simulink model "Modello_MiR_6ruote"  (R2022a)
settings: Solver=VariableStepAuto  StartTime=0.0  StopTime=time_v(end,1)  RelTol=1e-3
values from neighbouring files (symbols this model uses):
  a = 0.250    (= 0.25)    [Modello_MiR_6ruote_script.m]    (also in Modello_MiR_2ruote_script.m; Modello_MiR_6ruote_validato_script.m; Modello_MiR_UR_script.m)
  Att_C = 0.005    [Modello_MiR_6ruote_script.m]
  b = 0.1875    [Modello_MiR_6ruote_script.m]    (also in Modello_MiR_2ruote_script.m; Modello_MiR_6ruote_validato_script.m; Modello_MiR_UR_script.m)
  b_caster = 0.07    [Modello_MiR_6ruote_script.m]    (also in Modello_MiR_2ruote_script.m; Modello_MiR_6ruote_validato_script.m; Modello_MiR_UR_script.m)
  bd = 0.205    [Modello_MiR_6ruote_script.m]    (also in Modello_MiR_2ruote_script.m; Modello_MiR_6ruote_validato_script.m; Modello_MiR_UR_script.m)
  F23fun = @(u) (mv*9.801/4)-u(7)    [Modello_MiR_6ruote_script.m]    (also in Modello_MiR_6ruote_validato_script.m = @(u) (mv*9.801/4)-(mv*h*u(5)+(mv*9.801/4)*(2*a-b_caster*(cos)
  F43fun = @(u) (1/(2*bd))*(mv*u(6)*h+u(7)*(2*bd-b_caster*(sin(u(3))+sin(u(4))))+u(8)*(2*bd-b_caster*(sin(u(1))+sin(u(2)))))    [Modello_MiR_6ruote_script.m]    (also in Modello_MiR_6ruote_validato_script.m = @(u) (1/(2*bd))*(mv*u(6)*h+((mv*h*u(5)+(mv*9.801/4)*(2*a-b_c)
  F63fun = @(u) (mv*h*u(5)+(mv*9.801/4)*(2*a-b_caster*(cos(u(1))+cos(u(2)))))/(4*a-b_caster*(cos(u(1))+cos(u(2)))+b_caster*(cos(u(3))+cos(u(4))))    [Modello_MiR_6ruote_script.m]    (also in Modello_MiR_6ruote_validato_script.m)
  fm_fun = @(u) (u <= -am2 | u >= am2)*0 + (u > -am2 && u <= -am1)*(- u * Mza/(am2 -am1) - Mza * am2/(am2 -am1)) +           + (u > -am1 && u <= am1)*(Mza*u/ am1) + (u > am1 && u < am2)*(Mza * u/(am1 -am2) - Mza * am2/(am1 - am2))    [Modello_MiR_6ruote_script.m]    (also in Modello_MiR_6ruote_validato_script.m = @(u) (u <= -am2 || u >= am2) * 0 + (u > -am2 && u <= -am1) *; Modello_MiR_UR_script.m = @(u) (u <= -am2 || u >= am2) * 0 + (u > -am2 && u <= -am1) *)
  Icw_1 = 1/2 * mcw * rc^2    (= 0.002004225735)    [Modello_MiR_6ruote_script.m]    (also in Modello_MiR_2ruote_script.m; Modello_MiR_6ruote_validato_script.m; Modello_MiR_UR_script.m)
  Icw_2 = 1/12 * mcw * ec^2 + 1/4 * mcw * rc^2    (= 0.00104098243873)    [Modello_MiR_6ruote_script.m]    (also in Modello_MiR_2ruote_script.m; Modello_MiR_6ruote_validato_script.m; Modello_MiR_UR_script.m)
  Idw_1 = 1/2 * mdw * rd^2    (= 0.00551836278784)    [Modello_MiR_6ruote_script.m]    (also in Modello_MiR_2ruote_script.m; Transfer_Function_Gol_Gcl.m = Inertia_vect(jj,1); Modello_MiR_6ruote_validato_script.m; Modello_MiR_UR_script.m)
  iMax = 20.7*1.1    (= 22.77)    [Modello_MiR_6ruote_script.m]    (also in Modello_MiR_2ruote_script.m; Modello_MiR_6ruote_validato_script.m; Modello_MiR_UR_script.m)
  Iv = mv * (l^2 + w^2)  / 12    (= 6.75343333333)    [Modello_MiR_6ruote_script.m]    (also in Modello_MiR_2ruote_script.m; Modello_MiR_6ruote_validato_script.m = 8.95033333333; Modello_MiR_UR_script.m)
  Kc = 0.15    [Modello_MiR_6ruote_script.m]    (also in Modello_MiR_2ruote_script.m; Modello_MiR_6ruote_validato_script.m; Modello_MiR_UR_script.m)
  Ki_i = 1    [Modello_MiR_6ruote_script.m]    (also in Modello_MiR_2ruote_script.m; Modello_MiR_6ruote_validato_script.m; Modello_MiR_UR_script.m)
  Ki_v = 1    [Modello_MiR_6ruote_script.m]    (also in Modello_MiR_2ruote_script.m; Modello_MiR_6ruote_validato_script.m; Modello_MiR_UR_script.m)
  kk = 0.00005    (= 5e-05)    [Modello_MiR_6ruote_script.m]    (also in Modello_MiR_2ruote_script.m; Modello_MiR_6ruote_validato_script.m; Modello_MiR_UR_script.m)
  Kp_i = 5    [Modello_MiR_6ruote_script.m]    (also in Modello_MiR_2ruote_script.m; Modello_MiR_6ruote_validato_script.m; Modello_MiR_UR_script.m)
  Kp_v = 5    [Modello_MiR_6ruote_script.m]    (also in Modello_MiR_2ruote_script.m; Modello_MiR_6ruote_validato_script.m; Modello_MiR_UR_script.m)
  kv = 1.5e-6    (= 1.5e-06)    [Modello_MiR_6ruote_script.m]    (also in Modello_MiR_2ruote_script.m; Modello_MiR_6ruote_validato_script.m; Modello_MiR_UR_script.m)
  L = R * tauE    (= 0.00181134822805)    [Modello_MiR_6ruote_script.m]    (also in Modello_MiR_2ruote_script.m; Modello_MiR_6ruote_validato_script.m; Modello_MiR_UR_script.m)
  mcw = rc^2 * pi * ec * rhopoliu + 1    (= 1.02616357632)    [Modello_MiR_6ruote_script.m]    (also in Modello_MiR_2ruote_script.m; Modello_MiR_6ruote_validato_script.m; Modello_MiR_UR_script.m)
  mv = 83    [Modello_MiR_6ruote_script.m]    (also in Modello_MiR_2ruote_script.m; Modello_MiR_6ruote_validato_script.m = 110; Modello_MiR_UR_script.m)
  Psi_start = pi/2    (= 1.57079632679)    [Modello_MiR_6ruote_script.m]    (also in Modello_MiR_6ruote_validato_script.m = psi_mir(1,1); Modello_MiR_UR_script.m = psi_mir(1,1))
  R = velMax * TorqueMax / (iMax)^2    (= 1.81134822805)    [Modello_MiR_6ruote_script.m]    (also in Modello_MiR_2ruote_script.m; Modello_MiR_6ruote_validato_script.m; Modello_MiR_UR_script.m)
  rap_rid = 10.167    [Modello_MiR_6ruote_script.m]    (also in Modello_MiR_2ruote_script.m; Modello_MiR_6ruote_validato_script.m; Modello_MiR_UR_script.m)
  rc = 0.125/2    (= 0.0625)    [Modello_MiR_6ruote_script.m]    (also in Modello_MiR_2ruote_script.m; Modello_MiR_6ruote_validato_script.m; Modello_MiR_UR_script.m)
  rd = 0.1    [Modello_MiR_6ruote_script.m]    (also in Modello_MiR_2ruote_script.m; Modello_MiR_6ruote_validato_script.m; Modello_MiR_UR_script.m)
  Sx = spline(x ,fl_fun(x),zx)    [Modello_MiR_6ruote_script.m]
  Sy = spline(x ,ft_fun(x),zy)    [Modello_MiR_6ruote_script.m]
  VaMax = Kc * velMax    (= 41.2443991527)    [Modello_MiR_6ruote_script.m]    (also in Modello_MiR_2ruote_script.m; Modello_MiR_6ruote_validato_script.m; Modello_MiR_UR_script.m)
  X_start = input('Inserire coordinata x iniziale')    [Modello_MiR_6ruote_script.m]    (also in Modello_MiR_2ruote_script.m; Modello_MiR_6ruote_validato_script.m = traj(1,1); Modello_MiR_UR_script.m = traj(1,1))
  Y_start = input('Inserire coordinata y iniziale')    [Modello_MiR_6ruote_script.m]    (also in Modello_MiR_2ruote_script.m; Modello_MiR_6ruote_validato_script.m = traj(1,2); Modello_MiR_UR_script.m = traj(1,2))
  zx = linspace(inferior,superi,10001)    [Modello_MiR_6ruote_script.m]
  zy = linspace(inferior,superi,10001)    [Modello_MiR_6ruote_script.m]
libraries: slpidlib x4
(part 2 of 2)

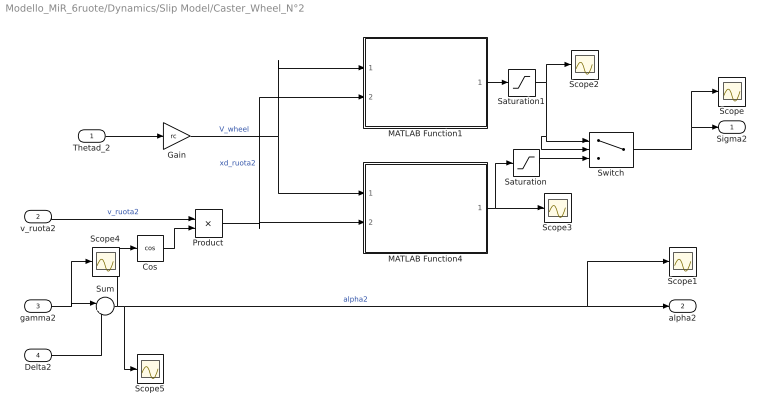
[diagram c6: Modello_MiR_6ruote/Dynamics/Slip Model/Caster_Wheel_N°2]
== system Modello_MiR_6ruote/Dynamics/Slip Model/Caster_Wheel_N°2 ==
  Thetad_2 : Inport
  v_ruota2 : Inport  Port=2
  gamma2 : Inport  Port=3
  Delta2 : Inport  Port=4
  Cos : Trigonometry  Operator=cos
  Gain : Gain  Gain=rc
  MATLAB Function1 : MATLAB Function  TreatAsAtomicUnit=on
  MATLAB Function4 : MATLAB Function  TreatAsAtomicUnit=on
  Product : Product
  Saturation : Saturate  UpperLimit=1  LowerLimit=-1
  Saturation1 : Saturate  UpperLimit=1  LowerLimit=-1
  Scope{,1..5} (6 alike) : Scope
  Sum : Sum  Inputs=|+-
  Switch : Switch
  Sigma2 : Outport
  alpha2 : Outport  Port=2
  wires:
  Thetad_2/1 -> Gain/1
  gamma2/1 -> Scope4/1, Sum/1
  Gain/1 -> MATLAB Function4/1(v_wheel), MATLAB Function1/1(v_wheel)  "V_wheel"
  Switch/1 -> Scope/1, Sigma2/1
  MATLAB Function1/1(Fc_pos_out) -> Saturation1/1
  MATLAB Function4/1(Fc_neg_out) -> Saturation/1, Scope3/1
  Product/1 -> MATLAB Function1/2(xd_ruota2), MATLAB Function4/2(xd_ruota2)  "xd_ruota2"
  v_ruota2/1 -> Product/1  "v_ruota2"
  Cos/1 -> Product/2
  Delta2/1 -> Sum/2
  Sum/1 -> Cos/1, Scope1/1, alpha2/1, Scope5/1  "alpha2"
  Saturation1/1 -> Scope2/1, Switch/2, Switch/1
  Saturation/1 -> Switch/3

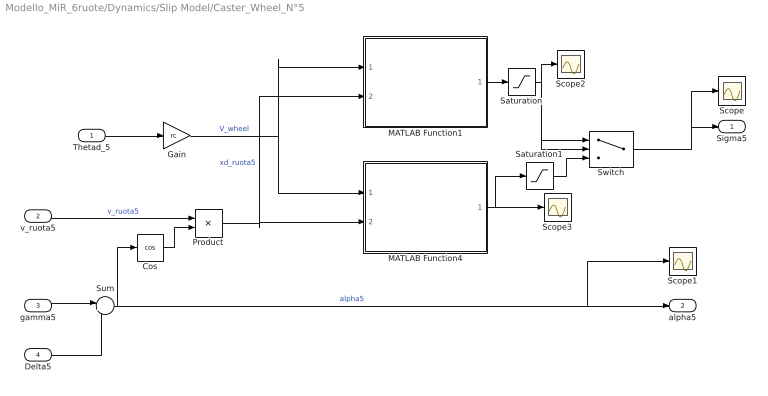
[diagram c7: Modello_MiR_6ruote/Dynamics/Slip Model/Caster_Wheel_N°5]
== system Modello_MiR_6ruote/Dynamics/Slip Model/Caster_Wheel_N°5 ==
  Thetad_5 : Inport
  v_ruota5 : Inport  Port=2
  gamma5 : Inport  Port=3
  Delta5 : Inport  Port=4
  Cos : Trigonometry  Operator=cos
  Gain : Gain  Gain=rc
  MATLAB Function1 : MATLAB Function  TreatAsAtomicUnit=on
  MATLAB Function4 : MATLAB Function  TreatAsAtomicUnit=on
  Product : Product
  Saturation : Saturate  UpperLimit=1  LowerLimit=-1
  Saturation1 : Saturate  UpperLimit=1  LowerLimit=-1
  Scope{,1..3} (4 alike) : Scope
  Sum : Sum  Inputs=|+-
  Switch : Switch
  Sigma5 : Outport
  alpha5 : Outport  Port=2
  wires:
  Thetad_5/1 -> Gain/1
  gamma5/1 -> Sum/1
  Gain/1 -> MATLAB Function4/1(v_wheel), MATLAB Function1/1(v_wheel)  "V_wheel"
  Switch/1 -> Scope/1, Sigma5/1
  MATLAB Function1/1(Fc_pos_out) -> Saturation/1
  MATLAB Function4/1(Fc_neg_out) -> Saturation1/1, Scope3/1
  Product/1 -> MATLAB Function1/2(xd_ruota5), MATLAB Function4/2(xd_ruota5)  "xd_ruota5"
  v_ruota5/1 -> Product/1  "v_ruota5"
  Cos/1 -> Product/2
  Delta5/1 -> Sum/2
  Sum/1 -> Scope1/1, alpha5/1, Cos/1  "alpha5"
  Saturation/1 -> Scope2/1, Switch/1, Switch/2
  Saturation1/1 -> Switch/3

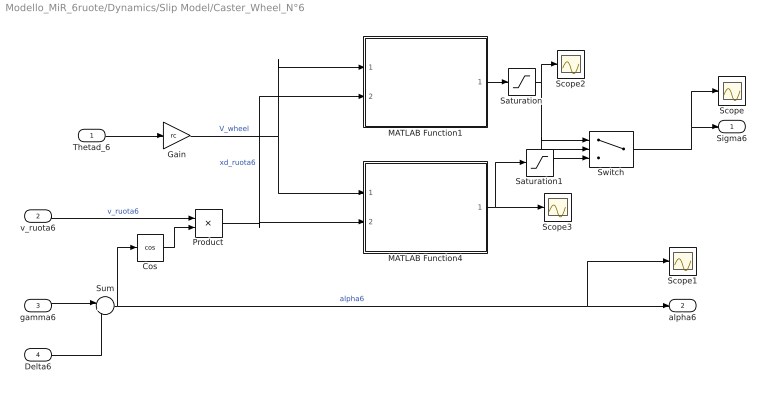
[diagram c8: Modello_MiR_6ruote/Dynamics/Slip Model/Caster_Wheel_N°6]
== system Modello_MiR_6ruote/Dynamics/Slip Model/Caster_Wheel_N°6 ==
  Thetad_6 : Inport
  v_ruota6 : Inport  Port=2
  gamma6 : Inport  Port=3
  Delta6 : Inport  Port=4
  Cos : Trigonometry  Operator=cos
  Gain : Gain  Gain=rc
  MATLAB Function1 : MATLAB Function  TreatAsAtomicUnit=on
  MATLAB Function4 : MATLAB Function  TreatAsAtomicUnit=on
  Product : Product
  Saturation : Saturate  UpperLimit=1  LowerLimit=-1
  Saturation1 : Saturate  UpperLimit=1  LowerLimit=-1
  Scope{,1..3} (4 alike) : Scope
  Sum : Sum  Inputs=|+-
  Switch : Switch
  Sigma6 : Outport
  alpha6 : Outport  Port=2
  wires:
  Thetad_6/1 -> Gain/1
  gamma6/1 -> Sum/1
  Gain/1 -> MATLAB Function4/1(v_wheel), MATLAB Function1/1(v_wheel)  "V_wheel"
  Switch/1 -> Scope/1, Sigma6/1
  MATLAB Function1/1(Fc_pos_out) -> Saturation/1
  MATLAB Function4/1(Fc_neg_out) -> Saturation1/1, Scope3/1
  Product/1 -> MATLAB Function1/2(xd_ruota6), MATLAB Function4/2(xd_ruota6)  "xd_ruota6"
  v_ruota6/1 -> Product/1  "v_ruota6"
  Cos/1 -> Product/2
  Delta6/1 -> Sum/2
  Sum/1 -> Scope1/1, alpha6/1, Cos/1  "alpha6"
  Saturation/1 -> Scope2/1, Switch/1, Switch/2
  Saturation1/1 -> Switch/3

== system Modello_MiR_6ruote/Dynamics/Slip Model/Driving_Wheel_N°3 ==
  Thetad_3 : Inport
  v_ruota3 : Inport  Port=2
  gamma3 : Inport  Port=3
  Gain : Gain  Gain=rd
  MATLAB Function1 : MATLAB Function  TreatAsAtomicUnit=on
  MATLAB Function4 : MATLAB Function  TreatAsAtomicUnit=on
  Saturation : Saturate  UpperLimit=1  LowerLimit=-1
  Saturation1 : Saturate  UpperLimit=1  LowerLimit=-1
  Scope{,1..4} (5 alike) : Scope
  Switch : Switch
  Sigma3 : Outport
  alpha3 : Outport  Port=2
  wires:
  Thetad_3/1 -> Gain/1
  Gain/1 -> MATLAB Function4/1(v_wheel), MATLAB Function1/1(v_wheel)  "V_wheel"
  Switch/1 -> Scope/1, Sigma3/1
  MATLAB Function1/1(Fc_pos_out) -> Saturation1/1
  MATLAB Function4/1(Fc_neg_out) -> Saturation/1, Scope3/1
  v_ruota3/1 -> MATLAB Function1/2(Vx_DL), MATLAB Function4/2(Vx_DL)  "xd_ruota3"
  Saturation1/1 -> Scope2/1, Switch/1, Switch/2
  Saturation/1 -> Switch/3
  gamma3/1 -> Scope1/1, alpha3/1, Scope4/1

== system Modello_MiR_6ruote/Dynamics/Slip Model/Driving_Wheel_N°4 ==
  Thetad_4 : Inport
  v_ruota4 : Inport  Port=2
  gamma4 : Inport  Port=3
  Gain : Gain  Gain=rd
  MATLAB Function1 : MATLAB Function  TreatAsAtomicUnit=on
  MATLAB Function4 : MATLAB Function  TreatAsAtomicUnit=on
  Saturation : Saturate  UpperLimit=1  LowerLimit=-1
  Saturation1 : Saturate  UpperLimit=1  LowerLimit=-1
  Scope{,1..4} (5 alike) : Scope
  Switch : Switch
  Sigma4 : Outport
  alpha4 : Outport  Port=2
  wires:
  Thetad_4/1 -> Gain/1
  Gain/1 -> MATLAB Function4/1(v_wheel), MATLAB Function1/1(v_wheel)  "V_wheel"
  Switch/1 -> Scope/1, Sigma4/1
  MATLAB Function1/1(Fc_pos_out) -> Saturation1/1
  MATLAB Function4/1(Fc_neg_out) -> Saturation/1
  v_ruota4/1 -> MATLAB Function1/2(Vx_DL), MATLAB Function4/2(Vx_DL)  "v_ruota4"
  Saturation1/1 -> Scope2/1, Switch/1, Switch/2
  Saturation/1 -> Switch/3, Scope3/1
  gamma4/1 -> Scope1/1, alpha4/1, Scope4/1

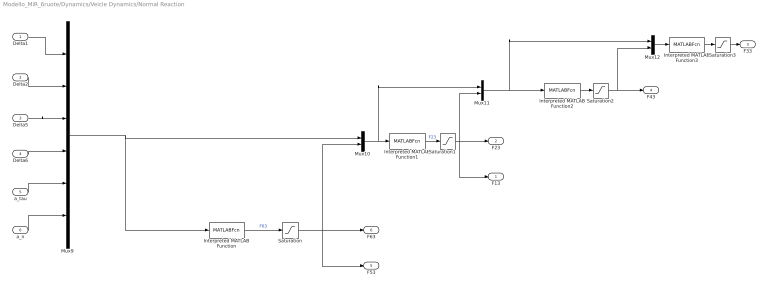
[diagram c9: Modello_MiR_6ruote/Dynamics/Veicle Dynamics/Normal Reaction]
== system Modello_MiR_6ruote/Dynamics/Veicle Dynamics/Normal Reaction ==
  Delta1 : Inport
  Delta2 : Inport  Port=2
  Delta5 : Inport  Port=3
  Delta6 : Inport  Port=4
  a_tau : Inport  Port=5
  a_n : Inport  Port=6
  Interpreted MATLAB Function : MATLABFcn  MATLABFcn=F63fun(u)
  Interpreted MATLAB Function1 : MATLABFcn  MATLABFcn=F23fun(u)
  Interpreted MATLAB Function2 : MATLABFcn  MATLABFcn=F43fun(u)
  Interpreted MATLAB Function3 : MATLABFcn  MATLABFcn=mv*9.801-2*u(7)-2*u(8)-u(9)
  Mux10 : Mux  Inputs=2
  Mux11 : Mux  Inputs=2
  Mux12 : Mux  Inputs=2
  Mux9 : Mux  Inputs=6
  Saturation{,1..3} (4 alike) : Saturate  UpperLimit=inf  LowerLimit=0
  F13 : Outport  PortDimensions=1
  F23 : Outport  Port=2  PortDimensions=1
  F33 : Outport  Port=3  PortDimensions=1
  F43 : Outport  Port=4  PortDimensions=1
  F53 : Outport  Port=5  PortDimensions=1
  F63 : Outport  Port=6  PortDimensions=1
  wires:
  Delta1/1 -> Mux9/1
  a_n/1 -> Mux9/6
  Mux10/1 -> Mux11/1, Interpreted MATLAB Function1/1
  Mux11/1 -> Interpreted MATLAB Function2/1, Mux12/1
  Delta6/1 -> Mux9/4
  Mux9/1 -> Mux10/1, Interpreted MATLAB Function/1
  Interpreted MATLAB Function3/1 -> Saturation3/1
  Mux12/1 -> Interpreted MATLAB Function3/1
  Delta5/1 -> Mux9/3
  a_tau/1 -> Mux9/5
  Interpreted MATLAB Function1/1 -> Saturation1/1  "F23"
  Delta2/1 -> Mux9/2
  Interpreted MATLAB Function/1 -> Saturation/1  "F63"
  Interpreted MATLAB Function2/1 -> Saturation2/1
  Saturation/1 -> F63/1, F53/1, Mux10/2
  Saturation1/1 -> F23/1, F13/1, Mux11/2
  Saturation2/1 -> F43/1, Mux12/2
  Saturation3/1 -> F33/1

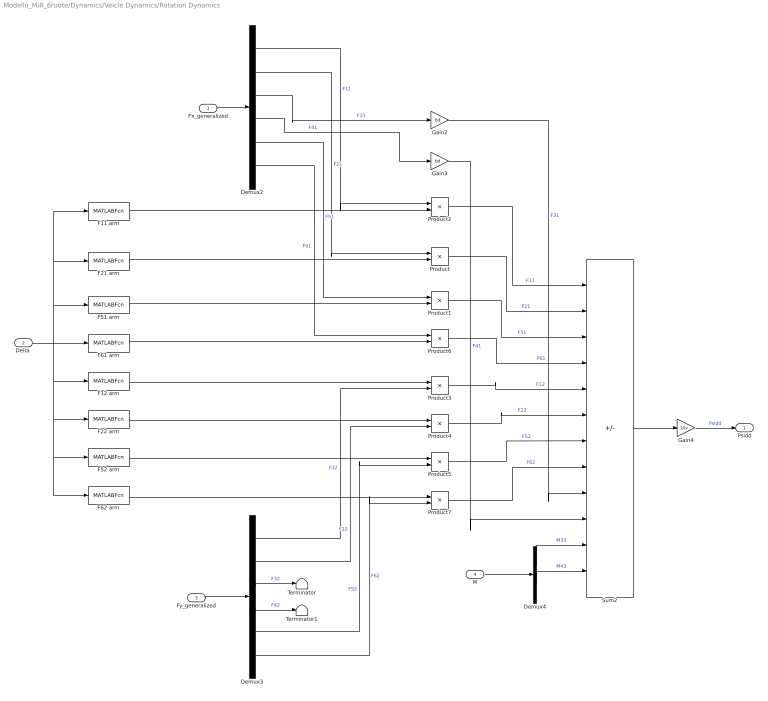
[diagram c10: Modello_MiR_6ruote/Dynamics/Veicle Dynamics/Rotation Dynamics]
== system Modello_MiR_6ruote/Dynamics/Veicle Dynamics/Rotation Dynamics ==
  Fx_generalized : Inport
  "Delta " : Inport  Port=2
  Fy_generalized : Inport  Port=3
  M : Inport  Port=4
  Demux2 : Demux  Outputs=6
  Demux3 : Demux  Outputs=6
  Demux4 : Demux  Outputs=2
  F11 arm : MATLABFcn  MATLABFcn=b-b_caster*sin(u(1))
  F12 arm : MATLABFcn  MATLABFcn=a-b_caster*cos(u(1))
  F21 arm : MATLABFcn  MATLABFcn=b+b_caster*sin(u(2))
  F22 arm : MATLABFcn  MATLABFcn=a-b_caster*cos(u(2))
  F51 arm : MATLABFcn  MATLABFcn=b-b_caster*sin(u(3))
  F52 arm : MATLABFcn  MATLABFcn=a+b_caster*cos(u(3))
  F61 arm : MATLABFcn  MATLABFcn=b+b_caster*sin(u(4))
  F62 arm : MATLABFcn  MATLABFcn=a+b_caster*cos(u(4))
  Gain2 : Gain  Gain=bd
  Gain3 : Gain  Gain=bd
  Gain4 : Gain  Gain=1/Iv
  Product{,1..7} (8 alike) : Product
  Sum2 : Sum  Inputs=-+-+++---+++
  Terminator : Terminator
  Terminator1 : Terminator
  Psidd : Outport  PortDimensions=1
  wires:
  Product2/1 -> Sum2/1  "F11"
  Demux3/2 -> Product4/2  "F22"
  Sum2/1 -> Gain4/1
  Demux3/3 -> Terminator/1  "F32"
  Product4/1 -> Sum2/6  "F22"
  Fx_generalized/1 -> Demux2/1
  Demux3/6 -> Product7/2  "F62"
  Demux2/2 -> Product/1  "F21"
  "Delta "/1 -> F51 arm/1, F21 arm/1, F11 arm/1, F62 arm/1, F52 arm/1, F22 arm/1, F12 arm/1, F61 arm/1
  Gain3/1 -> Sum2/10  "F41"
  Product7/1 -> Sum2/8  "F62"
  Gain2/1 -> Sum2/9  "F31"
  Product3/1 -> Sum2/5  "F12"
  Demux4/1 -> Sum2/11  "M33"
  Demux3/4 -> Terminator1/1  "F42"
  Demux4/2 -> Sum2/12  "M43"
  Demux2/1 -> Product2/1  "F11"
  Product/1 -> Sum2/2  "F21"
  Gain4/1 -> Psidd/1  "Psidd"
  Demux2/3 -> Gain2/1  "F31"
  Demux2/4 -> Gain3/1  "F41"
  F51 arm/1 -> Product1/2
  Demux3/5 -> Product5/2  "F52"
  F61 arm/1 -> Product6/2
  Demux2/5 -> Product1/1  "F51"
  Product5/1 -> Sum2/7  "F52"
  F21 arm/1 -> Product/2
  Demux3/1 -> Product3/2  "F12"
  Product1/1 -> Sum2/3  "F51"
  Demux2/6 -> Product6/1  "F61"
  F11 arm/1 -> Product2/2
  Product6/1 -> Sum2/4  "F61"
  Fy_generalized/1 -> Demux3/1
  M/1 -> Demux4/1
  F22 arm/1 -> Product4/1
  F52 arm/1 -> Product5/1
  F62 arm/1 -> Product7/1
  F12 arm/1 -> Product3/1

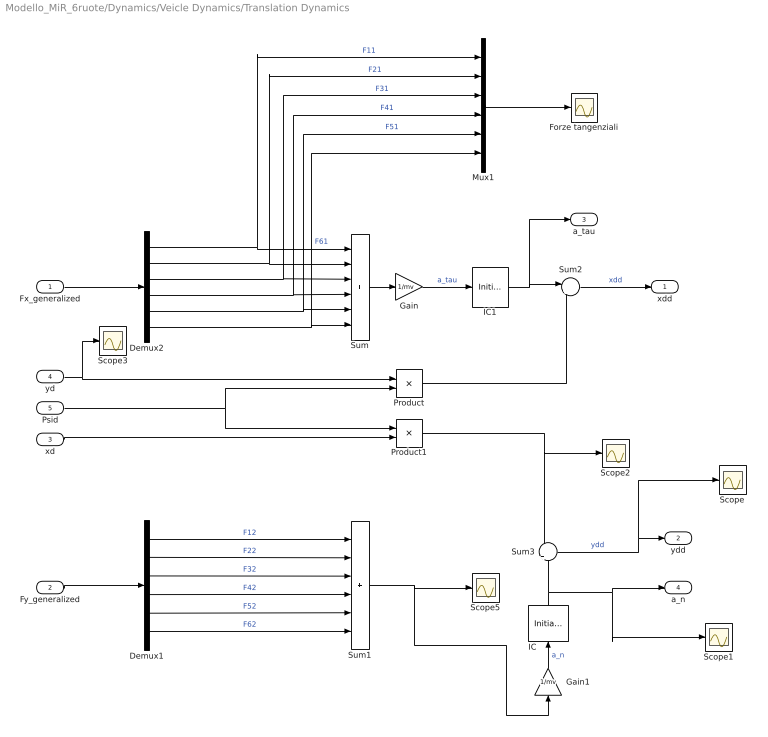
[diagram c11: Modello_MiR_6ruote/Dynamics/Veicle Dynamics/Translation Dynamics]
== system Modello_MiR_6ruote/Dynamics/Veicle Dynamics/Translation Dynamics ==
  Fx_generalized : Inport
  Fy_generalized : Inport  Port=2
  xd : Inport  Port=3
  yd : Inport  Port=4
  Psid : Inport  Port=5
  Demux1 : Demux  Outputs=6
  Demux2 : Demux  Outputs=6
  Forze tangenziali : Scope
  Gain : Gain  Gain=1/mv
  Gain1 : Gain  Gain=1/mv
  IC : InitialCondition  Value=0
  IC1 : InitialCondition  Value=0
  Mux1 : Mux  Inputs=6
  Product : Product
  Product1 : Product
  Scope{,1..3,5} (5 alike) : Scope
  Sum : Sum  Inputs=6
  Sum1 : Sum  Inputs=6
  Sum2 : Sum  Inputs=|++
  Sum3 : Sum  Inputs=-|+
  xdd : Outport  PortDimensions=1
  ydd : Outport  Port=2  PortDimensions=1
  a_tau : Outport  Port=3  PortDimensions=1
  a_n : Outport  Port=4  PortDimensions=1
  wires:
  Demux1/1 -> Sum1/1  "F12"
  Demux1/2 -> Sum1/2  "F22"
  Sum3/1 -> Scope/1, ydd/1  "ydd"
  Demux1/3 -> Sum1/3  "F32"
  Demux2/4 -> Mux1/4, Sum/4  "F41"
  Demux2/5 -> Mux1/5, Sum/5  "F51"
  Fx_generalized/1 -> Demux2/1
  Demux2/2 -> Sum/2, Mux1/2  "F21"
  Demux1/4 -> Sum1/4  "F42"
  Demux2/3 -> Sum/3, Mux1/3  "F31"
  Sum2/1 -> xdd/1  "xdd"
  Demux2/1 -> Sum/1, Mux1/1  "F11"
  Demux1/5 -> Sum1/5  "F52"
  Demux2/6 -> Mux1/6, Sum/6  "F61"
  Demux1/6 -> Sum1/6  "F62"
  Fy_generalized/1 -> Demux1/1
  Sum/1 -> Gain/1
  yd/1 -> Scope3/1, Product/1
  Psid/1 -> Product1/1, Product/2
  Gain/1 -> IC1/1  "a_tau"
  Product/1 -> Sum2/2
  xd/1 -> Product1/2
  Gain1/1 -> IC/1  "a_n"
  Product1/1 -> Scope2/1, Sum3/1
  Sum1/1 -> Gain1/1, Scope5/1
  Mux1/1 -> Forze tangenziali/1
  IC/1 -> Sum3/2, Scope1/1, a_n/1
  IC1/1 -> Sum2/1, a_tau/1

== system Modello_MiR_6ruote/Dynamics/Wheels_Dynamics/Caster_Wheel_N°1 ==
  Sigma1 : Inport
  alpha1 : Inport  Port=2
  F13 : Inport  Port=3
  Slip Forces/Torque : Subsystem
  Wheel Dynamics : Subsystem
  F1L : Outport
  F1T : Outport  Port=2
  Thetad_1 : Outport  Port=3
  Phid_1 : Outport  Port=4
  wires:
  Slip Forces/Torque/1(F1L) -> Wheel Dynamics/1(F1L), F1L/1  "F1L"
  alpha1/1 -> Slip Forces/Torque/2(Alpha1)
  Slip Forces/Torque/2(F1T) -> F1T/1
  Wheel Dynamics/2(Phid_1) -> Phid_1/1
  Sigma1/1 -> Slip Forces/Torque/1(Sigma1)
  Slip Forces/Torque/3(M13) -> Wheel Dynamics/2(M13)
  Wheel Dynamics/1(Thetad_1) -> Thetad_1/1
  F13/1 -> Wheel Dynamics/3(F13), Slip Forces/Torque/3(F13)

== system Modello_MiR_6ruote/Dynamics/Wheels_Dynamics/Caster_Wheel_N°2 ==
  Sigma2 : Inport
  alpha2 : Inport  Port=2
  F23 : Inport  Port=3
  Slip Forces/Torque : Subsystem
  Wheel Dynamics : Subsystem
  F2L : Outport
  F2T : Outport  Port=2
  Thetad_2 : Outport  Port=3
  Phid_2 : Outport  Port=4
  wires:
  Slip Forces/Torque/1(F2L) -> Wheel Dynamics/1(F2L), F2L/1
  alpha2/1 -> Slip Forces/Torque/2(Alpha2)
  Slip Forces/Torque/2(F2T) -> F2T/1
  Wheel Dynamics/2(Phid_2) -> Phid_2/1
  Sigma2/1 -> Slip Forces/Torque/1(Sigma2)
  Slip Forces/Torque/3(M23) -> Wheel Dynamics/2(M23)
  Wheel Dynamics/1(Thetad_2) -> Thetad_2/1
  F23/1 -> Wheel Dynamics/3(F23), Slip Forces/Torque/3(F23)

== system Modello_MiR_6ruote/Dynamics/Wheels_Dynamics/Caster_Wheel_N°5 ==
  Sigma5 : Inport
  alpha5 : Inport  Port=2
  F53 : Inport  Port=3
  Slip Forces/Torque : Subsystem
  Wheel Dynamics : Subsystem
  F5L : Outport
  F5T : Outport  Port=2
  Thetad_5 : Outport  Port=3
  Phid_5 : Outport  Port=4
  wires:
  alpha5/1 -> Slip Forces/Torque/2(Alpha5)
  Slip Forces/Torque/2(F5T) -> F5T/1
  Wheel Dynamics/2(Phid_5) -> Phid_5/1
  Sigma5/1 -> Slip Forces/Torque/1(Sigma5)
  Slip Forces/Torque/3(M53) -> Wheel Dynamics/2(M53)
  Wheel Dynamics/1(Thetad_5) -> Thetad_5/1
  F53/1 -> Wheel Dynamics/3(F53), Slip Forces/Torque/3(F53)
  Slip Forces/Torque/1(F5L) -> Wheel Dynamics/1(F5L), F5L/1

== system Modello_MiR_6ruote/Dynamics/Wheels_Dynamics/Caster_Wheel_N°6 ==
  Sigma6 : Inport
  alpha6 : Inport  Port=2
  F63 : Inport  Port=3
  Slip Forces/Torque : Subsystem
  Wheel Dynamics : Subsystem
  F6L : Outport
  F6T : Outport  Port=2
  Thetad_6 : Outport  Port=3
  Phid_6 : Outport  Port=4
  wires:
  Slip Forces/Torque/1(F6L) -> Wheel Dynamics/1(F6L), F6L/1
  alpha6/1 -> Slip Forces/Torque/2(Alpha6)
  Slip Forces/Torque/2(F6T) -> F6T/1
  Wheel Dynamics/2(Phid_6) -> Phid_6/1
  Sigma6/1 -> Slip Forces/Torque/1(Sigma6)
  Slip Forces/Torque/3(M63) -> Wheel Dynamics/2(M63)
  Wheel Dynamics/1(Thetad_6) -> Thetad_6/1
  F63/1 -> Wheel Dynamics/3(F63), Slip Forces/Torque/3(F63)

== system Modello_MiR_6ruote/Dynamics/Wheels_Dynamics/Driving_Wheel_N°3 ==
  Cm3 : Inport
  Sigma3 : Inport  Port=2
  alpha3 : Inport  Port=3
  F33 : Inport  Port=4
  Scope : Scope
  Scope1 : Scope
  Scope2 : Scope
  Subsystem : Subsystem
  Wheel Dynamics : Subsystem
  F3L : Outport
  F3T : Outport  Port=2
  M33 : Outport  Port=3
  Thetad_3 : Outport  Port=4
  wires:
  Cm3/1 -> Wheel Dynamics/1(Cm3)
  Wheel Dynamics/1(Thetad_3) -> Thetad_3/1
  Sigma3/1 -> Subsystem/1(Sigma3)
  alpha3/1 -> Subsystem/2(alpha3)
  Subsystem/1(F3L) -> Scope/1, F3L/1, Wheel Dynamics/2(F3L)  "F3L"
  Subsystem/2(F3T) -> F3T/1, Scope2/1  "F3T"
  Subsystem/3(M33) -> Scope1/1, M33/1
  F33/1 -> Wheel Dynamics/3(F33), Subsystem/3(F33)

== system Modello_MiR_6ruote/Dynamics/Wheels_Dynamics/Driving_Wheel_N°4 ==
  Cm4 : Inport
  Sigma4 : Inport  Port=2
  alpha4 : Inport  Port=3
  F43 : Inport  Port=4
  Scope : Scope
  Scope1 : Scope
  Scope2 : Scope
  Subsystem : Subsystem
  Subsystem1 : Subsystem
  F4L : Outport
  F4T : Outport  Port=2
  M43 : Outport  Port=3
  Thetad_4 : Outport  Port=4
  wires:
  Cm4/1 -> Subsystem/1(Cm4)
  alpha4/1 -> Subsystem1/2(alpha4)
  Sigma4/1 -> Subsystem1/1(Sigma4)
  Subsystem1/1(F4L) -> Scope/1, F4L/1, Subsystem/2(F4L)
  Subsystem1/2(F4T) -> Scope1/1, F4T/1
  Subsystem1/3(M43) -> Scope2/1, M43/1
  Subsystem/1(Thetad_4) -> Thetad_4/1
  F43/1 -> Subsystem/3(F43), Subsystem1/3(F43)

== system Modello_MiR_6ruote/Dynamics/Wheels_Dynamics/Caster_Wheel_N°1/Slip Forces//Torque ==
  Sigma1 : Inport
  Alpha1 : Inport  Port=2
  F13 : Inport  Port=3
  1-D Lookup Table : Lookup_n-D  NumberOfTableDimensions=1  BreakpointsForDimension1=zx  Table=Sx  InternalRulePriority=Speed  RndMeth=Simplest
  1-D Lookup Table1 : Lookup_n-D  NumberOfTableDimensions=1  BreakpointsForDimension1=zy  Table=Sy  InternalRulePriority=Speed  RndMeth=Simplest
  Gain : Gain  Gain=-1
  Interpreted MATLAB Function3 : MATLABFcn  MATLABFcn=u*b_caster
  Product : Product
  Product1 : Product
  Scope : Scope
  Scope1 : Scope
  F1L : Outport  PortDimensions=1
  F1T : Outport  Port=2
  M13 : Outport  Port=3
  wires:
  F13/1 -> Product1/2, Product/2
  Product/1 -> F1L/1, Scope/1  "F1L"
  Product1/1 -> Gain/1
  Alpha1/1 -> 1-D Lookup Table1/1
  Interpreted MATLAB Function3/1 -> M13/1
  Gain/1 -> F1T/1, Interpreted MATLAB Function3/1, Scope1/1
  Sigma1/1 -> 1-D Lookup Table/1
  1-D Lookup Table/1 -> Product/1
  1-D Lookup Table1/1 -> Product1/1

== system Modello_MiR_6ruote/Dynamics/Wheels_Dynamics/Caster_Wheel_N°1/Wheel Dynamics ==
  F1L : Inport
  M13 : Inport  Port=2
  F13 : Inport  Port=3
  Gain : Gain  Gain=-rc
  Gain1 : Gain  Gain=1/Icw_1
  Gain2 : Gain  Gain=1/(Icw_2+mcw*b_caster^2)
  Gain3 : Gain  Gain=Att_C
  Integrator : Integrator
  Integrator1 : Integrator
  Interpreted MATLAB Function : MATLABFcn  MATLABFcn=u(2)*(kk*u(1)+kv*u(1)^2)  OutputDimensions=1
  Mux : Mux  Inputs=2
  Mux1 : Mux  Inputs=2
  Scope : Scope
  Scope1 : Scope
  Scope2 : Scope
  Sum : Sum  Inputs=+-
  Sum1 : Sum  Inputs=--
  Thetad_1 : Outport
  Phid_1 : Outport  Port=2
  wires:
  Integrator/1 -> Mux/1, Thetad_1/1
  Sum/1 -> Scope/1, Gain1/1
  Gain1/1 -> Integrator/1
  F1L/1 -> Gain/1
  Gain/1 -> Sum/1
  Interpreted MATLAB Function/1 -> Sum/2
  M13/1 -> Sum1/1, Mux1/1  "M13"
  Sum1/1 -> Gain2/1
  Gain2/1 -> Integrator1/1
  Gain3/1 -> Mux1/2, Sum1/2  "Coppia_Attr"
  Mux/1 -> Interpreted MATLAB Function/1
  F13/1 -> Mux/2
  Mux1/1 -> Scope2/1
  Integrator1/1 -> Gain3/1, Scope1/1, Phid_1/1

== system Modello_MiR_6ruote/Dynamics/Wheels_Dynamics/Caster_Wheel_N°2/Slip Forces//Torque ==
  Sigma2 : Inport
  Alpha2 : Inport  Port=2
  F23 : Inport  Port=3
  1-D Lookup Table : Lookup_n-D  NumberOfTableDimensions=1  BreakpointsForDimension1=zx  Table=Sx  InternalRulePriority=Speed  RndMeth=Simplest
  1-D Lookup Table1 : Lookup_n-D  NumberOfTableDimensions=1  BreakpointsForDimension1=zy  Table=Sy  InternalRulePriority=Speed  RndMeth=Simplest
  Gain : Gain  Gain=-1
  Interpreted MATLAB Function3 : MATLABFcn  MATLABFcn=b_caster*u
  Product : Product
  Product1 : Product
  Scope : Scope
  F2L : Outport
  F2T : Outport  Port=2
  M23 : Outport  Port=3
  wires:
  Product1/1 -> Gain/1
  Gain/1 -> Interpreted MATLAB Function3/1, F2T/1
  Sigma2/1 -> 1-D Lookup Table/1
  Alpha2/1 -> 1-D Lookup Table1/1
  Interpreted MATLAB Function3/1 -> M23/1
  Product/1 -> F2L/1, Scope/1  "F1L"
  F23/1 -> Product1/2, Product/2
  1-D Lookup Table1/1 -> Product1/1
  1-D Lookup Table/1 -> Product/1

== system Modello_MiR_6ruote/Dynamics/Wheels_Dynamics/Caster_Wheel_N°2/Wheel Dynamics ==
  F2L : Inport
  M23 : Inport  Port=2
  F23 : Inport  Port=3
  Gain : Gain  Gain=-rc
  Gain1 : Gain  Gain=1/Icw_1
  Gain2 : Gain  Gain=1/(Icw_2+mcw*b_caster^2)
  Gain3 : Gain  Gain=Att_C
  Integrator : Integrator
  Integrator1 : Integrator
  Interpreted MATLAB Function : MATLABFcn  MATLABFcn=u(2)*(kk*u(1)+kv*u(1)^2)  OutputDimensions=1
  Mux : Mux  Inputs=2
  Mux1 : Mux  Inputs=2
  Scope : Scope
  Scope2 : Scope
  Sum : Sum  Inputs=+-
  Sum1 : Sum  Inputs=--
  Thetad_2 : Outport
  Phid_2 : Outport  Port=2
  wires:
  Integrator/1 -> Mux/1, Thetad_2/1
  Sum/1 -> Scope/1, Gain1/1
  Gain1/1 -> Integrator/1
  F2L/1 -> Gain/1
  Gain/1 -> Sum/1
  Interpreted MATLAB Function/1 -> Sum/2
  Sum1/1 -> Gain2/1
  Gain2/1 -> Integrator1/1
  Mux/1 -> Interpreted MATLAB Function/1
  F23/1 -> Mux/2
  Gain3/1 -> Mux1/2, Sum1/2  "Coppia_Attr"
  Mux1/1 -> Scope2/1
  M23/1 -> Sum1/1, Mux1/1  "M23"
  Integrator1/1 -> Gain3/1, Phid_2/1

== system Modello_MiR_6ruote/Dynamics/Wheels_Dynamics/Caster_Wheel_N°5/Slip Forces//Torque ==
  Sigma5 : Inport
  Alpha5 : Inport  Port=2
  F53 : Inport  Port=3
  1-D Lookup Table : Lookup_n-D  NumberOfTableDimensions=1  BreakpointsForDimension1=zx  Table=Sx  InternalRulePriority=Speed  RndMeth=Simplest
  1-D Lookup Table1 : Lookup_n-D  NumberOfTableDimensions=1  BreakpointsForDimension1=zy  Table=Sy  InternalRulePriority=Speed  RndMeth=Simplest
  Gain : Gain  Gain=-1
  Interpreted MATLAB Function3 : MATLABFcn  MATLABFcn=b_caster*u
  Product : Product
  Product1 : Product
  F5L : Outport
  F5T : Outport  Port=2
  M53 : Outport  Port=3
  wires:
  Product1/1 -> Gain/1
  Gain/1 -> Interpreted MATLAB Function3/1, F5T/1
  Interpreted MATLAB Function3/1 -> M53/1
  Product/1 -> F5L/1  "F1L"
  1-D Lookup Table1/1 -> Product1/1
  1-D Lookup Table/1 -> Product/1
  Alpha5/1 -> 1-D Lookup Table1/1
  Sigma5/1 -> 1-D Lookup Table/1
  F53/1 -> Product1/2, Product/2

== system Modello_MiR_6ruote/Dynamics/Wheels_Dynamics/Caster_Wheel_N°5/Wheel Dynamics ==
  F5L : Inport
  M53 : Inport  Port=2
  F53 : Inport  Port=3
  Gain : Gain  Gain=-rc
  Gain1 : Gain  Gain=1/Icw_1
  Gain2 : Gain  Gain=1/(Icw_2+mcw*b_caster^2)
  Gain3 : Gain  Gain=Att_C
  Integrator : Integrator
  Integrator1 : Integrator
  Interpreted MATLAB Function : MATLABFcn  MATLABFcn=u(2)*(kk*u(1)+kv*u(1)^2)  OutputDimensions=1
  Mux : Mux  Inputs=2
  Mux1 : Mux  Inputs=2
  Scope : Scope
  Scope2 : Scope
  Sum : Sum  Inputs=+-
  Sum1 : Sum  Inputs=--
  Thetad_5 : Outport
  Phid_5 : Outport  Port=2
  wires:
  Integrator/1 -> Mux/1, Thetad_5/1
  Sum/1 -> Scope/1, Gain1/1
  Gain1/1 -> Integrator/1
  F5L/1 -> Gain/1
  Gain/1 -> Sum/1
  Interpreted MATLAB Function/1 -> Sum/2
  Sum1/1 -> Gain2/1
  Gain2/1 -> Integrator1/1
  Mux/1 -> Interpreted MATLAB Function/1
  F53/1 -> Mux/2
  Gain3/1 -> Mux1/2, Sum1/2  "Coppia_Attr"
  Mux1/1 -> Scope2/1
  M53/1 -> Sum1/1, Mux1/1  "M53"
  Integrator1/1 -> Gain3/1, Phid_5/1

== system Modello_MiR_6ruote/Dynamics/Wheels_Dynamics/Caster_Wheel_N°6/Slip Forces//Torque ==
  Sigma6 : Inport
  Alpha6 : Inport  Port=2
  F63 : Inport  Port=3
  1-D Lookup Table : Lookup_n-D  NumberOfTableDimensions=1  BreakpointsForDimension1=zx  Table=Sx  InternalRulePriority=Speed  RndMeth=Simplest
  1-D Lookup Table1 : Lookup_n-D  NumberOfTableDimensions=1  BreakpointsForDimension1=zy  Table=Sy  InternalRulePriority=Speed  RndMeth=Simplest
  Gain : Gain  Gain=-1
  Interpreted MATLAB Function1 : MATLABFcn  MATLABFcn=b_caster*u
  Product : Product
  Product1 : Product
  F6L : Outport  PortDimensions=1
  F6T : Outport  Port=2  PortDimensions=1
  M63 : Outport  Port=3  PortDimensions=1
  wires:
  Product1/1 -> Gain/1
  Gain/1 -> Interpreted MATLAB Function1/1, F6T/1
  Interpreted MATLAB Function1/1 -> M63/1
  1-D Lookup Table1/1 -> Product1/1
  1-D Lookup Table/1 -> Product/1
  Product/1 -> F6L/1  "F1L"
  F63/1 -> Product1/2, Product/2
  Alpha6/1 -> 1-D Lookup Table1/1
  Sigma6/1 -> 1-D Lookup Table/1

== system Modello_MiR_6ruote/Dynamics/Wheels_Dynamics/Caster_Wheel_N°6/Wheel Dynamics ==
  F6L : Inport
  M63 : Inport  Port=2
  F63 : Inport  Port=3
  Gain : Gain  Gain=-rc
  Gain1 : Gain  Gain=1/Icw_1
  Gain2 : Gain  Gain=1/(Icw_2+mcw*b_caster^2)
  Gain3 : Gain  Gain=Att_C
  Integrator : Integrator
  Integrator1 : Integrator
  Interpreted MATLAB Function : MATLABFcn  MATLABFcn=u(2)*(kk*u(1)+kv*u(1)^2)  OutputDimensions=1
  Mux : Mux  Inputs=2
  Mux1 : Mux  Inputs=2
  Scope : Scope
  Scope2 : Scope
  Sum : Sum  Inputs=+-
  Sum1 : Sum  Inputs=--
  Thetad_6 : Outport
  Phid_6 : Outport  Port=2
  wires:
  Integrator/1 -> Mux/1, Thetad_6/1
  Sum/1 -> Scope/1, Gain1/1
  Gain1/1 -> Integrator/1
  F6L/1 -> Gain/1
  Gain/1 -> Sum/1
  Interpreted MATLAB Function/1 -> Sum/2
  Sum1/1 -> Gain2/1
  Gain2/1 -> Integrator1/1
  Mux/1 -> Interpreted MATLAB Function/1
  F63/1 -> Mux/2
  Gain3/1 -> Mux1/2, Sum1/2  "Coppia_Attr"
  Mux1/1 -> Scope2/1
  M63/1 -> Sum1/1, Mux1/1  "M63"
  Integrator1/1 -> Gain3/1, Phid_6/1

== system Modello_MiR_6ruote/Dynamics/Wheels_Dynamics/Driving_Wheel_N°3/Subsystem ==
  Sigma3 : Inport
  alpha3 : Inport  Port=2
  F33 : Inport  Port=3
  1-D Lookup Table : Lookup_n-D  NumberOfTableDimensions=1  BreakpointsForDimension1=zx  Table=Sx  InternalRulePriority=Speed  RndMeth=Simplest
  1-D Lookup Table1 : Lookup_n-D  NumberOfTableDimensions=1  BreakpointsForDimension1=zy  Table=Sy  InternalRulePriority=Speed  RndMeth=Simplest
  Gain : Gain  Gain=-1
  Interpreted MATLAB Function1 : MATLABFcn  MATLABFcn=fm_fun(u)  OutputDimensions=1
  Product : Product
  Product1 : Product
  Product2 : Product
  F3L : Outport
  F3T : Outport  Port=2
  M33 : Outport  Port=3
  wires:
  Gain/1 -> F3T/1
  F33/1 -> Product2/2, Product1/2, Product/2
  alpha3/1 -> 1-D Lookup Table1/1, Interpreted MATLAB Function1/1
  Product1/1 -> Gain/1
  Product/1 -> F3L/1  "F1L"
  1-D Lookup Table1/1 -> Product1/1
  1-D Lookup Table/1 -> Product/1
  Sigma3/1 -> 1-D Lookup Table/1
  Interpreted MATLAB Function1/1 -> Product2/1
  Product2/1 -> M33/1

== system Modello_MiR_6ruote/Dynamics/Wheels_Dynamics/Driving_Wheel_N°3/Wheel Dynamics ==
  Cm3 : Inport
  F3L : Inport  Port=2
  F33 : Inport  Port=3
  Gain : Gain  Gain=rd
  Gain1 : Gain  Gain=1/(Idw_1+2*10^(-3))
  Integrator : Integrator
  Interpreted MATLAB Function : MATLABFcn  MATLABFcn=u(2)*(kk*u(1)+kv*u(1)^2)  OutputDimensions=1
  Mux : Mux  Inputs=2
  Scope : Scope
  Scope1 : Scope
  Sum : Sum  Inputs=+--
  Thetad_3 : Outport
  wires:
  Cm3/1 -> Sum/1
  Gain/1 -> Scope1/1, Sum/2
  Interpreted MATLAB Function/1 -> Sum/3
  Integrator/1 -> Mux/1, Thetad_3/1
  Sum/1 -> Scope/1, Gain1/1
  Gain1/1 -> Integrator/1
  F3L/1 -> Gain/1
  Mux/1 -> Interpreted MATLAB Function/1
  F33/1 -> Mux/2

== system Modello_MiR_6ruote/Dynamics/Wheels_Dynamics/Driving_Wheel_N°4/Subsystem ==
  Cm4 : Inport
  F4L : Inport  Port=2
  F43 : Inport  Port=3
  Gain : Gain  Gain=rd
  Gain1 : Gain  Gain=1/(Idw_1+2*10^(-3))
  Integrator : Integrator
  Interpreted MATLAB Function : MATLABFcn  MATLABFcn=u(2)*(kk*u(1)+kv*u(1)^2)  OutputDimensions=1
  Mux : Mux  Inputs=3
  Mux1 : Mux  Inputs=2
  Scope : Scope
  Sum : Sum  Inputs=+--
  Thetad_4 : Outport
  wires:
  Interpreted MATLAB Function/1 -> Mux/2, Sum/3  "Res_rot"
  Gain/1 -> Mux/3, Sum/2  "rd*Fc_R"
  Sum/1 -> Gain1/1
  Gain1/1 -> Integrator/1
  Integrator/1 -> Mux1/1, Thetad_4/1
  F4L/1 -> Gain/1
  Cm4/1 -> Mux/1, Sum/1  "Cm_R"
  Mux/1 -> Scope/1
  Mux1/1 -> Interpreted MATLAB Function/1
  F43/1 -> Mux1/2

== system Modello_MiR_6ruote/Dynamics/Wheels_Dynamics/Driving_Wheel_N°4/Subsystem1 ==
  Sigma4 : Inport
  alpha4 : Inport  Port=2
  F43 : Inport  Port=3
  1-D Lookup Table : Lookup_n-D  NumberOfTableDimensions=1  BreakpointsForDimension1=zx  Table=Sx  InternalRulePriority=Speed  RndMeth=Simplest
  1-D Lookup Table1 : Lookup_n-D  NumberOfTableDimensions=1  BreakpointsForDimension1=zy  Table=Sy  InternalRulePriority=Speed  RndMeth=Simplest
  Gain : Gain  Gain=-1
  Interpreted MATLAB Function1 : MATLABFcn  MATLABFcn=fm_fun(u)  OutputDimensions=1
  Product : Product
  Product1 : Product
  Product2 : Product
  F4L : Outport
  F4T : Outport  Port=2
  M43 : Outport  Port=3
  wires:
  Gain/1 -> F4T/1
  F43/1 -> Product2/2, Product/2, Product1/2
  alpha4/1 -> Interpreted MATLAB Function1/1, 1-D Lookup Table1/1
  Product1/1 -> Gain/1
  Product/1 -> F4L/1  "F1L"
  1-D Lookup Table1/1 -> Product1/1
  1-D Lookup Table/1 -> Product/1
  Sigma4/1 -> 1-D Lookup Table/1
  Product2/1 -> M43/1
  Interpreted MATLAB Function1/1 -> Product2/1

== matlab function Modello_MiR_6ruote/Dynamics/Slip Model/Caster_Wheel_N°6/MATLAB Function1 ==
function Fc_pos_out = fcn(v_wheel,xd_ruota6)
x=v_wheel;
y=xd_ruota6;
cccc=1e20;

Fc_pos=@(x,y) ((((x-y)/abs(x+1/cccc))*(((x-y)/abs(x+1/cccc))<=1 )+ 1*(((x-y)/abs(x+1/cccc))>1))*(x*y>=0 && x>=0) + (((x-y)/abs(y+1/cccc))*(((x-y)/abs(y+1/cccc))<=1 ))*(x*y>0 && x<0)+ (x*y<0)*(x/abs(x+1/cccc)))*(0.02<(x^2+y^2)) + (10*(x-y)*(10*(x-y)<1) +1*(10*(x-y)>=1))*(0.02>=(x^2+y^2));

Fc_pos_out = Fc_pos(x,y);

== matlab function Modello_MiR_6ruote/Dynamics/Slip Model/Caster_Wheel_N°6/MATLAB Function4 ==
function Fc_neg_out = fcn(v_wheel,xd_ruota6)
x=v_wheel;
y=xd_ruota6;
cccc=1e20;

Fc_neg=@(x,y) ((((x-y)/abs(y+1/cccc))*(((x-y)/abs(y+1/cccc))>=-1)+ (-1)*(((x-y)/abs(y+1/cccc))<-1))*(x*y>=0 && y>=0) + (((x-y)/abs(x+1/cccc))*(((x-y)/abs(x+1/cccc))>=-1))*(x*y>0 && y<0) + (x*y<0)*(x/abs(x+1/cccc)) )*(0.02<(x^2+y^2)) +(10*(x-y)*(10*(x-y)>-1) -1*(10*(x-y)<=-1))*(0.02>=(x^2+y^2)); 

Fc_neg_out = Fc_neg(x,y);

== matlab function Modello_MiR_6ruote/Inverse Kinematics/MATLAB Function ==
function Thetad_DR_SET = angvelR(psi_set, Xd_set, Yd_set, psid_set)
 bd = 0.2050;
 rd = 0.1;
Thetad_DR_SET = 1/rd * (Xd_set * cos(psi_set) + Yd_set * sin(psi_set) + bd*psid_set);

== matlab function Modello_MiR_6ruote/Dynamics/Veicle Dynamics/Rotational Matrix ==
function [Fx_generalized, Fy_generalized] = fcn(FL,FT,Delta)
Fx_generalized=ones(6,1);
Fy_generalized=ones(6,1);

Fx_generalized(1,1)=FL(1)*cos(Delta(1))-FT(1)*sin(Delta(1));
Fy_generalized(1,1)=FT(1)*cos(Delta(1))+FL(1)*sin(Delta(1));
Fx_generalized(2,1)=FL(2)*cos(Delta(2))-FT(2)*sin(Delta(2));
Fy_generalized(2,1)=FT(2)*cos(Delta(2))+FL(2)*sin(Delta(2));
Fx_generalized(3,1)=FL(3);
Fy_generalized(3,1)=FT(3);
Fx_generalized(4,1)=FL(4);
Fy_generalized(4,1)=FT(4);
Fx_generalized(5,1)=FL(5)*cos(Delta(3))-FT(5)*sin(Delta(3));
Fy_generalized(5,1)=FT(5)*cos(Delta(3))+FL(5)*sin(Delta(3));
Fx_generalized(6,1)=FL(6)*cos(Delta(4))-FT(6)*sin(Delta(4));
Fy_generalized(6,1)=FT(6)*cos(Delta(4))+FL(6)*sin(Delta(4));

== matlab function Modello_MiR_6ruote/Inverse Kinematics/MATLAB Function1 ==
function Thetad_DL_SET = angvelL(psi_set, Xd_set, Yd_set, psid_set)
 bd = 0.2050;
 rd = 0.1;
Thetad_DL_SET = 1/rd * (Xd_set * cos(psi_set) + Yd_set * sin(psi_set) - bd*psid_set);

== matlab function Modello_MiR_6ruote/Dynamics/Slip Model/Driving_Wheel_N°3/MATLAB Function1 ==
function Fc_pos_out = fcn(v_wheel,Vx_DL)
x=v_wheel;
y=Vx_DL;
cccc=1e20;

Fc_pos=@(x,y) ((((x-y)/abs(x+1/cccc))*(((x-y)/abs(x+1/cccc))<=1 )+ 1*(((x-y)/abs(x+1/cccc))>1))*(x*y>=0 && x>=0) + (((x-y)/abs(y+1/cccc))*(((x-y)/abs(y+1/cccc))<=1 ))*(x*y>0 && x<0)+ (x*y<0)*(x/abs(x+1/cccc)))*(0.02<(x^2+y^2)) + (10*(x-y)*(10*(x-y)<1) +1*(10*(x-y)>=1))*(0.02>=(x^2+y^2));

Fc_pos_out = Fc_pos(x,y);

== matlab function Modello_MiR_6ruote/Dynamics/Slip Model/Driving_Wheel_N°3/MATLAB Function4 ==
function Fc_neg_out = fcn(v_wheel,Vx_DL)
x=v_wheel;
y=Vx_DL;
cccc=1e20;

Fc_neg=@(x,y) ((((x-y)/abs(y+1/cccc))*(((x-y)/abs(y+1/cccc))>=-1)+ (-1)*(((x-y)/abs(y+1/cccc))<-1))*(x*y>=0 && y>=0) + (((x-y)/abs(x+1/cccc))*(((x-y)/abs(x+1/cccc))>=-1))*(x*y>0 && y<0) + (x*y<0)*(x/abs(x+1/cccc)) )*(0.02<(x^2+y^2)) +(10*(x-y)*(10*(x-y)>-1) -1*(10*(x-y)<=-1))*(0.02>=(x^2+y^2)); 
Fc_neg_out = Fc_neg(x,y);

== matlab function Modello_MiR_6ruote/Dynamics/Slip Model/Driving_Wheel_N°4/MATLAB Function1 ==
function Fc_pos_out = fcn(v_wheel,Vx_DL)
x=v_wheel;
y=Vx_DL;
cccc=1e20;

Fc_pos=@(x,y) ((((x-y)/abs(x+1/cccc))*(((x-y)/abs(x+1/cccc))<=1 )+ 1*(((x-y)/abs(x+1/cccc))>1))*(x*y>=0 && x>=0) + (((x-y)/abs(y+1/cccc))*(((x-y)/abs(y+1/cccc))<=1 ))*(x*y>0 && x<0)+ (x*y<0)*(x/abs(x+1/cccc)))*(0.02<(x^2+y^2)) + (10*(x-y)*(10*(x-y)<1) +1*(10*(x-y)>=1))*(0.02>=(x^2+y^2));

Fc_pos_out = Fc_pos(x,y);

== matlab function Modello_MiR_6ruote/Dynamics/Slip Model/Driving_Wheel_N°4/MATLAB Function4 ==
function Fc_neg_out = fcn(v_wheel,Vx_DL)
x=v_wheel;
y=Vx_DL;
cccc=1e20;

Fc_neg=@(x,y) ((((x-y)/abs(y+1/cccc))*(((x-y)/abs(y+1/cccc))>=-1)+ (-1)*(((x-y)/abs(y+1/cccc))<-1))*(x*y>=0 && y>=0) + (((x-y)/abs(x+1/cccc))*(((x-y)/abs(x+1/cccc))>=-1))*(x*y>0 && y<0) + (x*y<0)*(x/abs(x+1/cccc)) )*(0.02<(x^2+y^2)) +(10*(x-y)*(10*(x-y)>-1) -1*(10*(x-y)<=-1))*(0.02>=(x^2+y^2)); 

Fc_neg_out = Fc_neg(x,y);

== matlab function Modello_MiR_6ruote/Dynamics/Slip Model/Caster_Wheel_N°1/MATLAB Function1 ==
function Fc_pos_out = fcn(v_wheel,xd_ruota1)
x=v_wheel;
y=xd_ruota1;
cccc=1e20;

Fc_pos=@(x,y) ((((x-y)/abs(x+1/cccc))*(((x-y)/abs(x+1/cccc))<=1 )+ 1*(((x-y)/abs(x+1/cccc))>1))*(x*y>=0 && x>=0) + (((x-y)/abs(y+1/cccc))*(((x-y)/abs(y+1/cccc))<=1 ))*(x*y>0 && x<0)+ (x*y<0)*(x/abs(x+1/cccc)))*(0.02<(x^2+y^2)) + (10*(x-y)*(10*(x-y)<1) +1*(10*(x-y)>=1))*(0.02>=(x^2+y^2));


Fc_pos_out = Fc_pos(x,y);

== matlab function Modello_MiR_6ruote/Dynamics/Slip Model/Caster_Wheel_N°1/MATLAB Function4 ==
function Fc_neg_out = fcn(v_wheel,xd_ruota1)
x=v_wheel;
y=xd_ruota1;
cccc=1e20;

Fc_neg=@(x,y) ((((x-y)/abs(y+1/cccc))*(((x-y)/abs(y+1/cccc))>=-1)+ (-1)*(((x-y)/abs(y+1/cccc))<-1))*(x*y>=0 && y>=0) + (((x-y)/abs(x+1/cccc))*(((x-y)/abs(x+1/cccc))>=-1))*(x*y>0 && y<0) + (x*y<0)*(x/abs(x+1/cccc)) )*(0.02<(x^2+y^2)) +(10*(x-y)*(10*(x-y)>-1) -1*(10*(x-y)<=-1))*(0.02>=(x^2+y^2)); 


Fc_neg_out = Fc_neg(x,y);

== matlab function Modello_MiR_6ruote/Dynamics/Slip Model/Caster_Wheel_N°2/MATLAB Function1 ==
function Fc_pos_out = fcn(v_wheel,xd_ruota2)
x=v_wheel;
y=xd_ruota2;
cccc=1e20;
Fc_pos=@(x,y) ((((x-y)/abs(x+1/cccc))*(((x-y)/abs(x+1/cccc))<=1 )+ 1*(((x-y)/abs(x+1/cccc))>1))*(x*y>=0 && x>=0) + (((x-y)/abs(y+1/cccc))*(((x-y)/abs(y+1/cccc))<=1 ))*(x*y>0 && x<0)+ (x*y<0)*(x/abs(x+1/cccc)))*(0.02<(x^2+y^2)) + (10*(x-y)*(10*(x-y)<1) +1*(10*(x-y)>=1))*(0.02>=(x^2+y^2));

Fc_pos_out = Fc_pos(x,y);

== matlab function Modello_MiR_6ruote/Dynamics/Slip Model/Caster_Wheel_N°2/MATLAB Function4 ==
function Fc_neg_out = fcn(v_wheel,xd_ruota2)
x=v_wheel;
y=xd_ruota2;
cccc=1e20;

Fc_neg=@(x,y) ((((x-y)/abs(y+1/cccc))*(((x-y)/abs(y+1/cccc))>=-1)+ (-1)*(((x-y)/abs(y+1/cccc))<-1))*(x*y>=0 && y>=0) + (((x-y)/abs(x+1/cccc))*(((x-y)/abs(x+1/cccc))>=-1))*(x*y>0 && y<0) + (x*y<0)*(x/abs(x+1/cccc)) )*(0.02<(x^2+y^2)) +(10*(x-y)*(10*(x-y)>-1) -1*(10*(x-y)<=-1))*(0.02>=(x^2+y^2)); 

Fc_neg_out = Fc_neg(x,y);

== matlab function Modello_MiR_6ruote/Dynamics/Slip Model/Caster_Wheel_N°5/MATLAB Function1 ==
function Fc_pos_out = fcn(v_wheel,xd_ruota5)
x=v_wheel;
y=xd_ruota5;
cccc=1e20;

Fc_pos=@(x,y) ((((x-y)/abs(x+1/cccc))*(((x-y)/abs(x+1/cccc))<=1 )+ 1*(((x-y)/abs(x+1/cccc))>1))*(x*y>=0 && x>=0) + (((x-y)/abs(y+1/cccc))*(((x-y)/abs(y+1/cccc))<=1 ))*(x*y>0 && x<0)+ (x*y<0)*(x/abs(x+1/cccc)))*(0.02<(x^2+y^2)) + (10*(x-y)*(10*(x-y)<1) +1*(10*(x-y)>=1))*(0.02>=(x^2+y^2));

Fc_pos_out = Fc_pos(x,y);

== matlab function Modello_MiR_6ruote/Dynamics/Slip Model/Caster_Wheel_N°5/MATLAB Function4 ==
function Fc_neg_out = fcn(v_wheel,xd_ruota5)
x=v_wheel;
y=xd_ruota5;
cccc=1e20;

Fc_neg=@(x,y) ((((x-y)/abs(y+1/cccc))*(((x-y)/abs(y+1/cccc))>=-1)+ (-1)*(((x-y)/abs(y+1/cccc))<-1))*(x*y>=0 && y>=0) + (((x-y)/abs(x+1/cccc))*(((x-y)/abs(x+1/cccc))>=-1))*(x*y>0 && y<0) + (x*y<0)*(x/abs(x+1/cccc)) )*(0.02<(x^2+y^2)) +(10*(x-y)*(10*(x-y)>-1) -1*(10*(x-y)<=-1))*(0.02>=(x^2+y^2)); 

Fc_neg_out = Fc_neg(x,y);
